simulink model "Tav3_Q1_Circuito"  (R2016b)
settings: Solver=ode23s  StartTime=0.0  StopTime=Ts  RelTol=1e-12  EnableMultiTasking=on
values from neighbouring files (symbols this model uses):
  C2 = zpk(-1/ans,[],1)    [PID_Sevilla.m]
undefined symbols (not defined in the file or in its folder): C4, L3, L5, R1, R6
libraries: fl_lib x7, nesl_utility x3, elec_lib x2

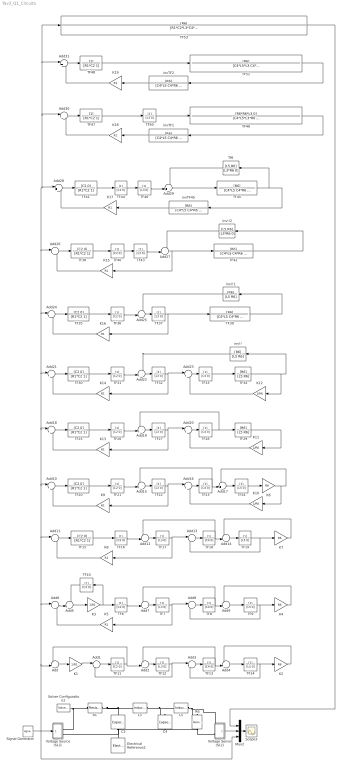
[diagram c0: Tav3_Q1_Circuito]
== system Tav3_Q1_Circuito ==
  Add{,2,4..5,7,9,12,14..15,17,19,22,25,27,29} (15 alike) : Sum  Inputs=-+|
  Add{1,3,6,8,10..11,13,16,18,20..21,23..24,26,28,30..31} (17 alike) : Sum  Inputs=|+-
  C2 : fl_lib/Electrical/Electrical Elements/Capacitor  c=C2 F  r=0 Ohm  g=0 1/Ohm  i_specify=off  i_priority=None  i=0 A  v_specify=off  v_priority=None  v=0 V  vc_specify=on  vc_priority=High  vc=0 V
  C4 : fl_lib/Electrical/Electrical Elements/Capacitor  c=C4 F  r=0 Ohm  g=0 1/Ohm  i_specify=off  i_priority=None  i=0 A  v_specify=off  v_priority=None  v=0 V  vc_specify=on  vc_priority=High  vc=0 V
  Electrical Reference2 : fl_lib/Electrical/Electrical Elements/Electrical Reference
  K1 : Gain  Gain=1/R1
  K10 : Gain  Gain=1/R6
  K11 : Gain  Gain=1/R6
  K12 : Gain  Gain=1/R6
  K{5,8..9,13..19} (10 alike) : Gain  Gain=R1
  K{2,4,6..7} (4 alike) : Gain  Gain=R6
  K3 : Gain  Gain=1/R1
  L3 : elec_lib/Passive Devices/Inductor  l=L3 H  L_tol=20  enable_L_tol=0  tol_distribution=1  nSigma=4  r=0 Ohm  g=1e-9 1/Ohm  initI=0 A  enable_operating_limits=0  operating_limit_action=2  max_working_current=1 A  power_rating=1 W  enable_faults=0  fault_action=1  lambdaPercent=50  k_faulted=0.9999 Ohm  turnsShort=0  openCct=0  groundShort=0  groundShortG=0 1/Ohm  tau_fault=0.001 s  enable_temporal_fault=0  t_fault=1 s  enable_behavioral_fault=0  max_permissible_voltage=100 V  n_fail_on_voltage=1  max_permissible_current=1 A  t_fail_on_current=1 s
  L5 : elec_lib/Passive Devices/Inductor  l=L5 H  L_tol=20  enable_L_tol=0  tol_distribution=1  nSigma=4  r=0 Ohm  g=1e-9 1/Ohm  initI=0 A  enable_operating_limits=0  operating_limit_action=2  max_working_current=1 A  power_rating=1 W  enable_faults=0  fault_action=1  lambdaPercent=50  k_faulted=0.9999 Ohm  turnsShort=0  openCct=0  groundShort=0  groundShortG=0 1/Ohm  tau_fault=0.001 s  enable_temporal_fault=0  t_fault=1 s  enable_behavioral_fault=0  max_permissible_voltage=100 V  n_fail_on_voltage=1  max_permissible_current=1 A  t_fail_on_current=1 s
  Mux2 : Mux  Inputs=3
  R1 : fl_lib/Electrical/Electrical Elements/Resistor  R=R1 Ohm  i_specify=off  i_priority=None  i=0 A  v_specify=off  v_priority=None  v=0 V
  R6 : fl_lib/Electrical/Electrical Elements/Resistor  R=R6 Ohm  i_specify=off  i_priority=None  i=0 A  v_specify=off  v_priority=None  v=0 V
  Scope3 : Scope
  Signal Generator : SignalGenerator  WaveForm=square
  Solver Configuration2 : nesl_utility/Solver Configuration  PhysicalDomain=network_engine_domain  SubClassName=solver  LeftPortType=input  RightPortType=generic  Accelerate=off  Tones=[]  Harmonics=[]  SimulateNoise=off  Profile=off  UseLocalSampling=off  EnableSwitchedLinearOptims=on  FrequencyDomain=off  UseCCode=off  RelTol=0.001  AbsTol=1e-06  MinStep=1e-09  ToWorkspace=off  RevertToSquareIcSolve=off  NumHomotopyIterations=100  PhasorMode=off  PhasorModeNumHarmonics=1  OverrideAbsTol=off  DoDC=off  ResidualTolerance=1e-6  UseLocalSolver=off  LocalSolverChoice=NE_TRAPEZOIDAL_ADVANCER  LocalSolverSampleTime=.0001  DoFixedCost=off  MaxNonlinIter=3  MaxModeIter=2  LinearAlgebra=Sparse  DelaysMemoryBudget=1024  AutomaticFiltering=on  FilteringTimeConstant=0.001
  TF{6,10..11,16,21,26,31,36,40,44} (10 alike) : TransferFcn  Denominator=[C2 0]
  TF{7,12,17,22,27,32,37,43,46,50} (10 alike) : TransferFcn  Denominator=[L3 0]
  TF{8,13,18,23,28,33} (6 alike) : TransferFcn  Denominator=[C4 0]
  TF{9,14,19,24} (4 alike) : TransferFcn  Denominator=[L5 0]
  TF{15,20,25,30,35,38,41} (7 alike) : TransferFcn  Numerator=[C2 0]  Denominator=[R1*C2 1]
  TF29 : TransferFcn  Numerator=[R6]  Denominator=[L5 R6]
  TF34 : TransferFcn  Numerator=[R6]  Denominator=[L5 R6]
  TF39 : TransferFcn  Numerator=[R6]  Denominator=[C4*L5 C4*R6 1]
  TF42 : TransferFcn  Numerator=[R6]  Denominator=[C4*L5 C4*R6 1]
  TF45 : TransferFcn  Numerator=[R6]  Denominator=[C4*L5 C4*R6 1]
  TF47 : TransferFcn  Denominator=[R1*C2 1]
  TF48 : TransferFcn  Denominator=[R1*C2 1]
  TF49 : TransferFcn  Numerator=[R6*R6*L3 0]  Denominator=[C4*L5*L3*R6 C4*R6*L3*R6 L3*R6+R6*L5 R6*R6]
  TF51 : TransferFcn  Numerator=[R6]  Denominator=[C4*L5*L3 C4*L3*R6 L3+L5 R6]
  TF53 : TransferFcn  Numerator=[R6]  Denominator="[R1*C2*L3*C4*L5   L3*C4*L5+R1*C2*L3*C4*R6   R1*C2*(L3+L5)+L3*C4*R6+R1*C4*L5 L3+L5+R1*R6*C2+R1*C4*R6  R1+R6]"
  Tf6 : TransferFcn  Numerator=[L5 R6]  Denominator=[L3*R6 0]
  Voltage Sensor (SL)1 : Subsystem
  Voltage Source (SL)1 : Subsystem
  inv!! : TransferFcn  Numerator=[R6]  Denominator=[L5 R6]
  inv!!1 : TransferFcn  Numerator=[R6]  Denominator=[L5 R6]
  inv!!2 : TransferFcn  Numerator=[L5 R6]  Denominator=[L3*R6 0]
  invTF1 : TransferFcn  Numerator=[R6]  Denominator=[C4*L5 C4*R6 1]
  invTF2 : TransferFcn  Numerator=[R6]  Denominator=[C4*L5 C4*R6 1]
  invTF45 : TransferFcn  Numerator=[R6]  Denominator=[C4*L5 C4*R6 1]
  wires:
  Mux2/1 -> Scope3/1
  Add/1 -> K1/1
  TF11/1 -> Add2/2, Add/1
  Add1/1 -> TF11/1
  Add2/1 -> TF12/1
  K1/1 -> Add1/1
  TF12/1 -> Add3/1, Add1/2
  Add3/1 -> TF13/1
  TF13/1 -> Add2/1, Add4/2
  Add4/1 -> TF14/1
  TF14/1 -> Add3/2, K2/1
  K2/1 -> Add4/1
  Voltage Sensor (SL)1/1(v) -> Mux2/2
  TF6/1 -> Add7/2
  Add7/1 -> TF7/1
  TF7/1 -> Add8/1, K5/1
  Add8/1 -> TF8/1
  TF8/1 -> Add7/1, Add9/2
  Add9/1 -> TF9/1
  TF9/1 -> Add8/2, K4/1
  K4/1 -> Add9/1
  TF10/1 -> Add5/1
  K3/1 -> TF10/1, TF6/1
  K5/1 -> Add6/2
  Add6/1 -> Add5/2
  Add5/1 -> K3/1
  TF16/1 -> Add12/2
  Add12/1 -> TF17/1
  TF17/1 -> Add13/1, K8/1
  Add13/1 -> TF18/1
  TF18/1 -> Add12/1, Add14/2
  Add14/1 -> TF19/1
  TF19/1 -> Add13/2, K7/1
  K7/1 -> Add14/1
  TF15/1 -> TF16/1
  K8/1 -> Add11/2
  Add11/1 -> TF15/1
  TF21/1 -> Add15/2
  Add15/1 -> TF22/1
  TF22/1 -> Add16/1, K9/1
  Add16/1 -> TF23/1
  TF23/1 -> Add15/1, Add17/2
  Add17/1 -> TF24/1
  TF24/1 -> K6/1
  TF20/1 -> TF21/1
  K9/1 -> Add10/2
  Add10/1 -> TF20/1
  K6/1 -> Add17/1, K10/1
  K10/1 -> Add16/2
  TF26/1 -> Add19/2
  Add19/1 -> TF27/1
  TF27/1 -> Add20/1, K13/1
  Add20/1 -> TF28/1
  TF28/1 -> TF29/1, Add19/1
  TF25/1 -> TF26/1
  K13/1 -> Add18/2
  Add18/1 -> TF25/1
  TF29/1 -> K11/1
  K11/1 -> Add20/2
  TF31/1 -> Add22/2
  Add22/1 -> TF32/1
  TF32/1 -> Add23/1, K14/1
  Add23/1 -> TF33/1
  TF33/1 -> TF34/1
  TF30/1 -> TF31/1
  K14/1 -> Add21/2
  Add21/1 -> TF30/1
  TF34/1 -> inv!!/1, K12/1
  K12/1 -> Add23/2
  inv!!/1 -> Add22/1
  TF36/1 -> Add25/2
  Add25/1 -> TF37/1
  TF37/1 -> TF39/1, K16/1
  TF35/1 -> TF36/1
  K16/1 -> Add24/2
  Add24/1 -> TF35/1
  TF39/1 -> inv!!1/1
  inv!!1/1 -> Add25/1
  TF40/1 -> TF43/1
  Add27/1 -> TF42/1, K15/1
  TF38/1 -> TF40/1
  K15/1 -> Add26/2
  Add26/1 -> TF38/1
  TF42/1 -> inv!!2/1
  TF43/1 -> Add27/2
  inv!!2/1 -> Add27/1
  TF44/1 -> TF46/1
  Add29/1 -> TF45/1
  TF41/1 -> TF44/1
  K17/1 -> Add28/2
  Add28/1 -> TF41/1
  TF45/1 -> invTF45/1, Tf6/1
  TF46/1 -> Add29/2
  Tf6/1 -> Add29/1
  invTF45/1 -> K17/1
  TF47/1 -> TF50/1
  TF50/1 -> TF49/1
  K18/1 -> Add30/2
  Add30/1 -> TF47/1
  TF49/1 -> invTF1/1
  invTF1/1 -> K18/1
  TF48/1 -> TF51/1
  K19/1 -> Add31/2
  Add31/1 -> TF48/1
  TF51/1 -> invTF2/1
  invTF2/1 -> K19/1
  Signal Generator/1 -> TF53/1, Add31/1, Add30/1, Add28/1, Add26/1, Add24/1, Add21/1, Add18/1, Add10/1, Add11/1, Add6/1, Add/2, Mux2/3, Voltage Source (SL)1/1(S)
  TF53/1 -> Mux2/1
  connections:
  R1/RConn1 -- C2/LConn1 -- L3/LConn1
  Voltage Source (SL)1/RConn1 -- R1/LConn1 -- Solver Configuration2/RConn1
  C4/RConn1 -- Electrical Reference2/LConn1 -- C2/RConn1 -- Voltage Source (SL)1/RConn2 -- R6/RConn1 -- Voltage Sensor (SL)1/LConn2
  L3/RConn1 -- L5/LConn1 -- C4/LConn1
  L5/RConn1 -- Voltage Sensor (SL)1/LConn1 -- R6/LConn1

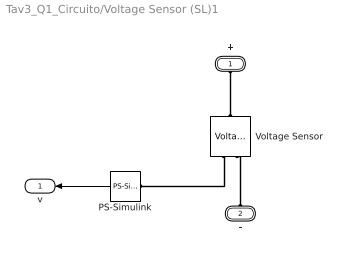
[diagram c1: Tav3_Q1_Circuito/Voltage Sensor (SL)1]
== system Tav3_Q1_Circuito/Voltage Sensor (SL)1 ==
  PS-Simulink : nesl_utility/PS-Simulink Converter  PhysicalDomain=network_engine_domain  SubClassName=ps_output  LeftPortType=input  RightPortType=output  PseudoPeriodic=off  Frequencies=[]  Unit=V  AffineConversion=off
  Voltage Sensor : fl_lib/Electrical/Electrical Sensors/Voltage Sensor
  + : PMIOPort  Port=1  Side=Left
  - : PMIOPort  Port=2  Side=Left
  v : Outport
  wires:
  PS-Simulink/1 -> v/1
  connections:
  Voltage Sensor/RConn1 -- PS-Simulink/LConn1
  +/RConn1 -- Voltage Sensor/LConn1
  -/RConn1 -- Voltage Sensor/RConn2

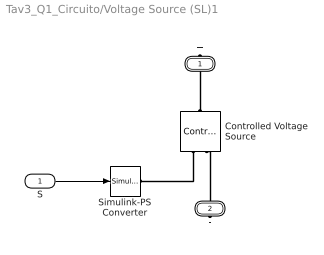
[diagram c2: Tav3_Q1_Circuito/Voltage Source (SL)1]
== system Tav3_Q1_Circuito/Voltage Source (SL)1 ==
  S : Inport
  Controlled Voltage Source : fl_lib/Electrical/Electrical Sources/Controlled Voltage Source
  Simulink-PS Converter : nesl_utility/Simulink-PS Converter  PhysicalDomain=network_engine_domain  SubClassName=ps_input  LeftPortType=input  RightPortType=output  PseudoPeriodic=off  Frequencies=[]  NoiseDistribution=none  NoiseParameters=[]  Unit=V  AffineConversion=off  InputFiltering=off  SimscapeFilterOrder=1  InputFilterTimeConstant=.001  UdotUserProvided=0
  + : PMIOPort  Port=1  Side=Right
  - : PMIOPort  Port=2  Side=Right
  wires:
  S/1 -> Simulink-PS Converter/1
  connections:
  Controlled Voltage Source/RConn1 -- Simulink-PS Converter/RConn1
  -/RConn1 -- Controlled Voltage Source/RConn2
  +/RConn1 -- Controlled Voltage Source/LConn1
